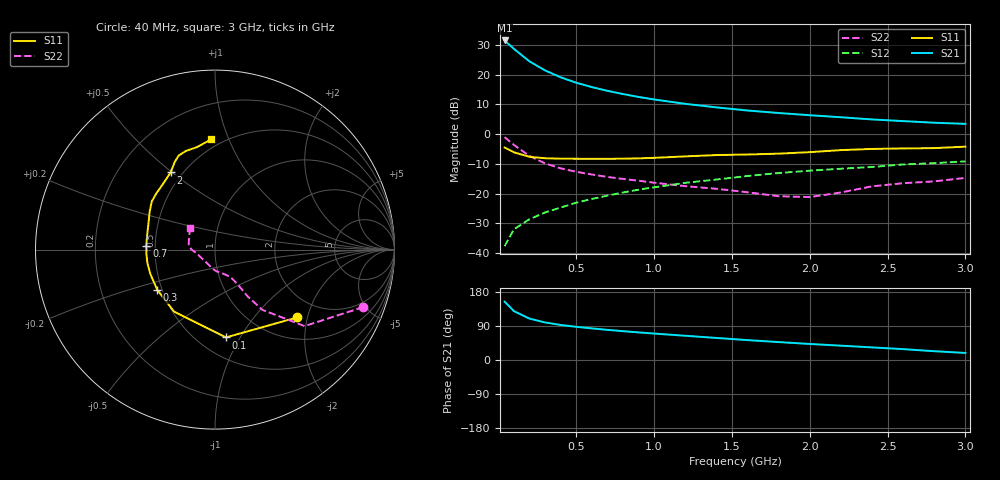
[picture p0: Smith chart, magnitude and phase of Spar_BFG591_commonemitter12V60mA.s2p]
! Filename:  BFG591F.S2P  Version:  4.0
! NXP part #: BFG591  Date: Jun 1994
! Bias condition: Vce=12V; Ic=60mA
#  MHz  S  MA  R  50
! Freq  S11  S21  S12  S22  !GUM [dB]
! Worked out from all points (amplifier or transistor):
!   21 points, 40 MHz to 3 GHz, reference 50 ohm
!   highest |S21| = 31.5 dB at 40 MHz (marker M1)
!   |S21| within 3 dB of that: start of sweep to 103.9 MHz
!   unconditionally stable (mu >= 1): 623.9 MHz to 2.199 GHz
!   at 300 MHz: K = 0.83, MSG = 23.9 dB, |S12| = -26.4 dB
!   at 1 GHz: K = 1.05, MAG = 13.4 dB, |S12| = -17.9 dB
!   at 3 GHz: K = 0.95, MSG = 6.3 dB, |S12| = -9.2 dB
!   S11 on the Smith chart (normalised r, x): 40 MHz: 1.48, -1.73; 100 MHz: 0.68, -0.87; 300 MHz: 0.47, -0.25; 700 MHz: 0.45, +0.02; 2 GHz: 0.43, +0.49; 3 GHz: 0.44, +0.86
40  0.594 -39.5  37.54 154.0  0.013 73.9  0.886 -21.2
100  0.493 -82.9  27.08 128.9  0.025 62.1  0.656 -40.5
200  0.414 -123.4  16.68 109.2  0.037 60.1  0.427 -51.8
300  0.392 -145.1  11.75 99.1  0.048 62.1  0.321 -55.0
400  0.385 -159.0  9.012 92.5  0.058 64.0  0.265 -56.0
500  0.384 -168.7  7.304 87.6  0.07 65.6  0.232 -56.9
600  0.383 -176.7  6.167 83.4  0.081 66.2  0.209 -58.0
700  0.383 176.6  5.336 79.6  0.092 66.7  0.19 -59.3
800  0.385 170.4  4.711 76.1  0.104 66.9  0.176 -61.0
900  0.39 164.2  4.213 72.8  0.116 66.9  0.164 -63.6
1000  0.398 158.7  3.815 69.8  0.127 66.5  0.152 -66.9
1200  0.421 149.8  3.225 64.0  0.151 65.4  0.133 -76.0
1400  0.443 142.7  2.811 58.2  0.172 63.4  0.12 -87.0
1600  0.453 135.9  2.49 52.5  0.197 62.3  0.105 -98.9
1800  0.468 127.9  2.261 47.3  0.221 59.3  0.09 -114.9
2000  0.496 119.9  2.073 42.3  0.242 57.5  0.087 -143.3
2200  0.537 114.7  1.918 37.8  0.261 55.3  0.104 -168.0
2400  0.562 111.1  1.762 33.3  0.279 54.3  0.132 179.4
2600  0.573 106.5  1.652 28.7  0.308 50.7  0.149 168.9
2800  0.58 99.8  1.551 23.2  0.324 46.8  0.16 155.0
3000  0.614 92.1  1.485 18.6  0.347 45.3  0.183 139.0
